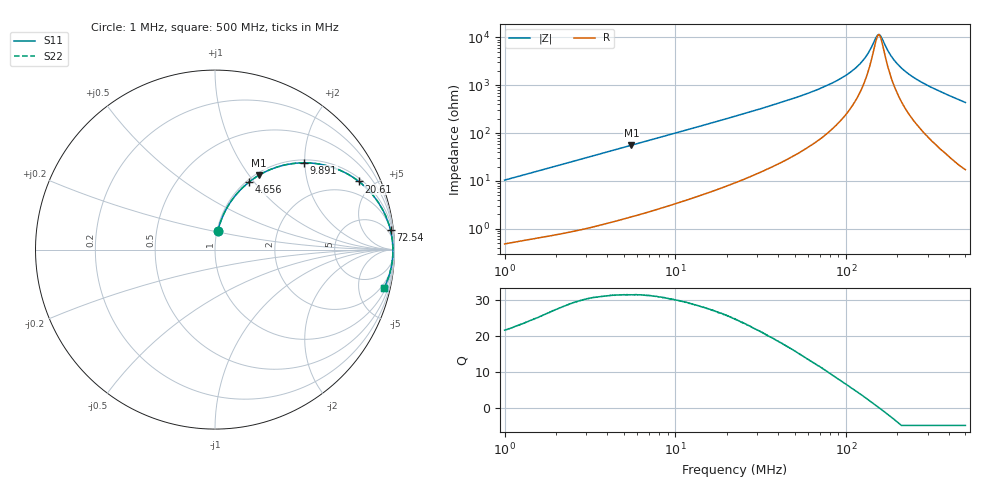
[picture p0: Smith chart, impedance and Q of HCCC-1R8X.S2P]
!s-Parameter Generated by FASTRON Sdn. Bhd.
!FASTRON P/N : HCCC-1R8X
!Keysight Technologies,E4991B,MY54100416,A.01.15
!Date: Thu Apr 02 13:59:03 2026
!Version  : Rev00 Thu Apr 02 13:59:03 2026
!Data & Calibration Information:
!PortZ  Port1:50+j0  Port2:50+j0
!When reading, reference impedance value at option line is always used.
! Remarks : This data is being provided solely for informational purposes.
!Freq	S11	S21	S12	S22
# Hz S dB R 50
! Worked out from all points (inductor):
!   1601 points, 1 MHz to 500 MHz, reference 50 ohm
!   read as one part in series: L = 1.64 uH near 1.032 MHz
!   highest Q = 31.5 at 5.524 MHz (marker M1), where L = 1.61 uH
!   self-resonance near 155.5 MHz
!   S11 on the Smith chart (normalised r, x): 1 MHz: 1.01, +0.21; 4.656 MHz: 1.03, +0.94; 9.891 MHz: 1.07, +1.98; 20.61 MHz: 1.16, +4.14; 72.54 MHz: 3, +18; 500 MHz: 1.35, -8.74
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1000000  -19.74 81.4  -0.09 -5.9  -0.09 -5.9  -19.74 81.4
2820919  -11.25 72.2  -0.42 -15.9  -0.42 -15.9  -11.25 72.2
4655808  -7.51 63.3  -0.98 -24.9  -0.98 -24.9  -7.51 63.3
5523530  -6.37 59.5  -1.29 -28.7  -1.29 -28.7  -6.37 59.5
7957584  -4.22 50.2  -2.28 -37.9  -2.28 -37.9  -4.22 50.2
9891114  -3.19 44.3  -3.12 -43.8  -3.12 -43.8  -3.19 44.3
2.060919e7  -1.04 25.3  -7.37 -62.4  -7.37 -62.4  -1.04 25.3
2.236068e7  -0.91 23.6  -7.96 -64.1  -7.96 -64.1  -0.91 23.6
3.577623e7  -0.42 14.9  -11.78 -72.2  -11.78 -72.2  -0.42 14.9
6.307767e7  -0.17 7.7  -17.46 -77.8  -17.46 -77.8  -0.17 7.7
7.254416e7  -0.14 6.3  -19.17 -78.5  -19.17 -78.5  -0.14 6.3
9.520996e7  -0.10 3.9  -23.36 -78.2  -23.36 -78.2  -0.10 3.9
1.160679e8  -0.09 2.3  -27.87 -74.9  -27.87 -74.9  -0.09 2.3
1.314291e8  -0.08 1.3  -32.33 -67.4  -32.33 -67.4  -0.08 1.3
1.494024e8  -0.08 0.3  -39.89 -31.3  -39.89 -31.3  -0.08 0.3
1.541177e8  -0.08 0.1  -41.17 -7.9  -41.17 -7.9  -0.08 0.1
1.608452e8  -0.08 -0.3  -40.24 27.6  -40.24 27.6  -0.08 -0.3
1.77937e8  -0.08 -1.0  -33.89 64.0  -33.89 64.0  -0.08 -1.0
2.054376e8  -0.08 -2.2  -28.11 75.4  -28.11 75.4  -0.08 -2.2
2.494725e8  -0.09 -3.9  -23.33 79.0  -23.33 79.0  -0.09 -3.9
3.325448e8  -0.14 -6.8  -18.50 79.1  -18.50 79.1  -0.14 -6.8
5e8  -0.29 -12.8  -13.12 75.0  -13.12 75.0  -0.29 -12.8
